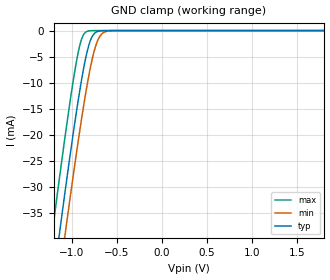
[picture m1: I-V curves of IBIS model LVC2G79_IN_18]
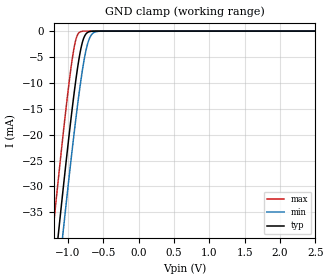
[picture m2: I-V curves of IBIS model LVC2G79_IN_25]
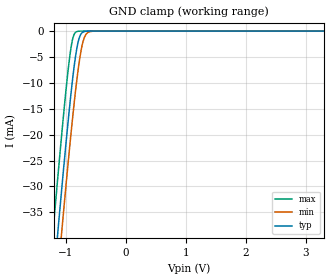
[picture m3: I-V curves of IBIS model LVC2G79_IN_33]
| TEXAS INSTRUMENTS INCORPORATED
| Standard Linear and Logic Group
| IBIS Model of SN74LVC2G79
| SINGLE-POSITIVE-EDGE-TRIGGERED D-TYPE FLIP-FLOP
| This file contains package information for the following:
|  SOT 8-pin (DCT) package as [Component] LVC2G79_DCT
|  SOT 8-pin (DCU) package as [Component] LVC2G79_DCU
|  DSBGA 8-pin (YEP) package as [Component] LVC2G79_YEP
|  DSBGA 8-pin (YZP) package as [Component] LVC2G79_YZP
| This device can be powered at the following Vccs:
|  1.8 volt Vcc
|  2.5 volt Vcc
|  3.3 volt Vcc
|  5 volt Vcc
| This file provides unique models under the [Model Selector] for each Vcc.
| For operation at a specific Vcc, select the appropriate model after each
| [Model Selector] keyword.
[IBIS Ver]   3.2
[Comment char]  |_char
[File Name]   sn74lvc2g79.ibs
[File Rev]   1.2 | d_die
[Date]   November 24, 2003
[Source]   Data created from TI-SPICE simulations at TI-SLL.
[Notes]   The following is an IBIS list for the LVC2G79.
   Please contact sllibis@ti.com with questions and
   comments concerning SLL IBIS models.
   - Due to the fact that the Device is 5.5-V Input tolarent,
   the pulldown model has some Non-Monotonic Warnings.
   - Power clamp data deleted as there is no power-clamp diode.
[Disclaimer] Property of Texas Instruments Incorporated.  Unauthorized
   reproduction and/or distribution is strictly prohibited.
   This product is protected under copyright law.
   Created  2003, (C) Copyright  2003, Texas Instruments
   Incorporated, All Rights Reserved
   UNLESS THERE IS A SIGNED, WRITTEN AGREEMENT TO THE
   CONTRARY, TEXAS INSTRUMENTS (TI) IS PROVIDING THE IBIS
   MODELS  AND WITHOUT ANY WARRANTY, EXPRESSED OR
   IMPLIED.  TI assumes no liability for:
   1) the accuracy of the IBIS models provided to your
   company;
   2) the proper functioning of these IBIS Models in your
   design or for any resulting applications; or
   3) infringement of patents, copyrights or intellectual
   property rights resulting from your use of these IBIS
   models.
   TI provides IBIS Models as a service to our customers.
   You and your company shall not distribute, sell or give
   these models to anyone else without prior written
   permission from TI.
   TI reserves the right to make changes to our products or
   to discontinue any semiconductor product or service
   without notice, and advises our customers to obtain the
   latest version of relevant information to verify, before
   placing orders, that the information being relied on is
   current.
   Please be aware that your receipt and use of the IBIS
   information provided shall serve as acceptance of these
   terms and conditions.  If you do not accept these terms,
   you should return or destroy the IBIS models and any
   other accompanying information immediately.
| Component LVC2G79_DCT 8-pin SOT
[Component]   LVC2G79_DCT
[Manufacturer]   Texas Instruments, Inc.
[Package]
|   typ   min   max
R_pkg   2.900e-02   2.800e-02   3.100e-02
L_pkg   1.796e-09   1.666e-09   1.924e-09
C_pkg   2.310e-13   2.210e-13   2.420e-13
[Pin]   signal_name   model_name   R_pin   L_pin   C_pin
1   1CLK   LVC2G79_IN   3.100e-02   1.894e-09   2.230e-13
2   1D   LVC2G79_IN   2.800e-02   1.697e-09   2.370e-13
3   2Q   LVC2G79_OUT   3.000e-02   1.722e-09   2.390e-13
4   GND   GND   3.000e-02   1.861e-09   2.210e-13
5   2CLK   LVC2G79_IN   2.800e-02   1.924e-09   2.280e-13
6   2D   LVC2G79_IN   2.900e-02   1.736e-09   2.420e-13
7   1Q   LVC2G79_OUT   2.800e-02   1.666e-09   2.360e-13
8   VCC   POWER   3.000e-02   1.871e-09   2.220e-13
| Component LVC2G79_DCU 8-pin SOT
[Component]   LVC2G79_DCU
[Manufacturer]   Texas Instruments, Inc.
[Package]
|   typ   min   max
R_pkg   2.600e-02   2.300e-02   3.800e-02
L_pkg   1.394e-09   1.066e-09   2.046e-09
C_pkg   2.590e-13   2.150e-13   3.720e-13
[Pin]   signal_name   model_name   R_pin   L_pin   C_pin
1   1CLK   LVC2G79_IN   2.400e-02   1.520e-09   2.710e-13
2   1D   LVC2G79_IN   2.300e-02   1.112e-09   2.180e-13
3   2Q   LVC2G79_OUT   2.300e-02   1.070e-09   2.170e-13
4   GND   GND   2.700e-02   2.046e-09   3.720e-13
5   2CLK   LVC2G79_IN   2.700e-02   1.542e-09   2.730e-13
6   2D   LVC2G79_IN   2.300e-02   1.100e-09   2.240e-13
7   1Q   LVC2G79_OUT   2.300e-02   1.066e-09   2.150e-13
8   VCC   POWER   3.800e-02   1.696e-09   2.800e-13
| Component LVC2G79_YEP 8-pin DSBGA
[Component]   LVC2G79_YEP
[Manufacturer]   Texas Instruments, Inc.
[Package]
|   typ   min   max
R_pkg   1.000e-03   1.000e-03   1.000e-03
L_pkg   2.450e-11   2.400e-11   2.500e-11
C_pkg   6.550e-14   6.400e-14   6.700e-14
[Pin]   signal_name   model_name   R_pin   L_pin   C_pin
1   1CLK   LVC2G79_IN   1.000e-03   2.500e-11   6.400e-14
2   1D   LVC2G79_IN   1.000e-03   2.400e-11   6.700e-14
3   2Q   LVC2G79_OUT   1.000e-03   2.400e-11   6.700e-14
4   GND   GND   1.000e-03   2.500e-11   6.400e-14
5   2CLK   LVC2G79_IN   1.000e-03   2.500e-11   6.400e-14
6   2D   LVC2G79_IN   1.000e-03   2.400e-11   6.700e-14
7   1Q   LVC2G79_OUT   1.000e-03   2.400e-11   6.700e-14
8   VCC   POWER   1.000e-03   2.500e-11   6.400e-14
| Component LVC2G79_YZP 8-pin DSBGA
[Component]   LVC2G79_YZP
[Manufacturer]   Texas Instruments, Inc.
[Package]
|   typ   min   max
R_pkg   1.000e-03   1.000e-03   1.000e-03
L_pkg   2.450e-11   2.400e-11   2.500e-11
C_pkg   6.550e-14   6.400e-14   6.700e-14
[Pin]   signal_name   model_name   R_pin   L_pin   C_pin
1   1CLK   LVC2G79_IN   1.000e-03   2.500e-11   6.400e-14
2   1D   LVC2G79_IN   1.000e-03   2.400e-11   6.700e-14
3   2Q   LVC2G79_OUT   1.000e-03   2.400e-11   6.700e-14
4   GND   GND   1.000e-03   2.500e-11   6.400e-14
5   2CLK   LVC2G79_IN   1.000e-03   2.500e-11   6.400e-14
6   2D   LVC2G79_IN   1.000e-03   2.400e-11   6.700e-14
7   1Q   LVC2G79_OUT   1.000e-03   2.400e-11   6.700e-14
8   VCC   POWER   1.000e-03   2.500e-11   6.400e-14
| Model LVC2G79_IN
[Model Selector]   LVC2G79_IN
LVC2G79_IN_18   1.8 volt Vcc
LVC2G79_IN_25   2.5 volt Vcc
LVC2G79_IN_33   3.3 volt Vcc
LVC2G79_IN_50   5 volt Vcc
| Model LVC2G79_OUT
[Model Selector]   LVC2G79_OUT
LVC2G79_OUT_18   1.8 volt Vcc
LVC2G79_OUT_25   2.5 volt Vcc
LVC2G79_OUT_33   3.3 volt Vcc
LVC2G79_OUT_50   5 volt Vcc
| Models and submodels in the file (8): LVC2G79_IN_18 (Input), LVC2G79_IN_25 (Input), LVC2G79_IN_33 (Input), LVC2G79_IN_50 (Input), LVC2G79_OUT_18 (Output), LVC2G79_OUT_25 (Output), LVC2G79_OUT_33 (Output), LVC2G79_OUT_50 (Output)
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[Model]   LVC2G79_IN_18
Model_type  Input
Vinl=0.5775
Vinh=1.2675
| variable   typ   min   max
C_comp   3.50pF   3.06pF   4.28pF
[Temperature Range]   40   100   -40
| Ambient temperature   25   85   -40
[Voltage range]   1.8   1.65   1.95
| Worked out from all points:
|   GND clamp passes 1 mA (typ) near -0.77 V on its own axis
[GND Clamp]
| LVC2G79_IN_18
|   Voltage   I(typ)   I(min)   I(max)
-5.5V     -655.2mA   -662.2mA   -646.6mA
-1.215V   -49.6mA    -57.88mA   -38.96mA
-1.135V   -39.07mA   -47.36mA   -28.42mA
-1.075V   -31.35mA   -39.6mA    -20.75mA
-1.055V   -28.82mA   -37.05mA   -18.27mA
-955mV    -16.68mA   -24.66mA   -6.874mA
-885mV    -9.098mA   -16.55mA   -1.486mA
-825mV    -3.922mA   -10.26mA   -137.1uA
-780mV    -1.472mA   -6.227mA   -17.15uA
-715mV    -205.4uA   -2.128mA   -808.5nA
-650mV    -22.01uA   -443.9uA   -37.93nA
1.8V      3.326pA    6.142pA    3.026pA
[Model]   LVC2G79_IN_25
Model_type  Input
Vinl=0.7
Vinh=1.7
| variable   typ   min   max
C_comp   3.42pF   2.84pF   4.36pF
[Temperature Range]   40   100   -40
| Ambient temperature   25   85   -40
[Voltage range]   2.5   2.3   2.7
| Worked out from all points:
|   GND clamp passes 1 mA (typ) near -0.77 V on its own axis
[GND Clamp]
| LVC2G79_IN_25
|   Voltage   I(typ)   I(min)   I(max)
-5.5V     -655.2mA   -662.2mA   -646.6mA
-1.215V   -49.6mA    -57.88mA   -38.96mA
-1.14V    -39.72mA   -48.01mA   -29.07mA
-1.12V    -37.12mA   -45.41mA   -26.48mA
-1.08V    -31.98mA   -40.25mA   -21.38mA
-1.06V    -29.44mA   -37.69mA   -18.89mA
-960mV    -17.26mA   -25.26mA   -7.377mA
-890mV    -9.597mA   -17.1mA    -1.734mA
-785mV    -1.671mA   -6.635mA   -21.67uA
-720mV    -242.5uA   -2.354mA   -1.023uA
-650mV    -22.01uA   -443.9uA   -37.93nA
2.5V      4.713pA    7.577pA    4.389pA
[Model]   LVC2G79_IN_33
Model_type  Input
Vinl=0.8
Vinh=2.0
| variable   typ   min   max
C_comp   3.35pF   2.69pF   4.41pF
[Temperature Range]   40   100   -40
| Ambient temperature   25   85   -40
[Voltage range]   3.3   3   3.6
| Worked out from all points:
|   GND clamp passes 1 mA (typ) near -0.77 V on its own axis
[GND Clamp]
| LVC2G79_IN_33
|   Voltage   I(typ)   I(min)   I(max)
-5.5V     -655.2mA   -662.2mA   -646.6mA
-1.225V   -50.93mA   -59.21mA   -40.3mA
-1.145V   -40.37mA   -48.66mA   -29.72mA
-1.12V    -37.12mA   -45.41mA   -26.48mA
-1.08V    -31.98mA   -40.25mA   -21.38mA
-1.06V    -29.44mA   -37.69mA   -18.89mA
-965mV    -17.84mA   -25.87mA   -7.89mA
-885mV    -9.098mA   -16.55mA   -1.486mA
-780mV    -1.472mA   -6.227mA   -17.15uA
-715mV    -205.4uA   -2.128mA   -808.5nA
-640mV    -15.53uA   -338.1uA   -23.69nA
3.3V      6.304pA    9.258pA    5.93pA
